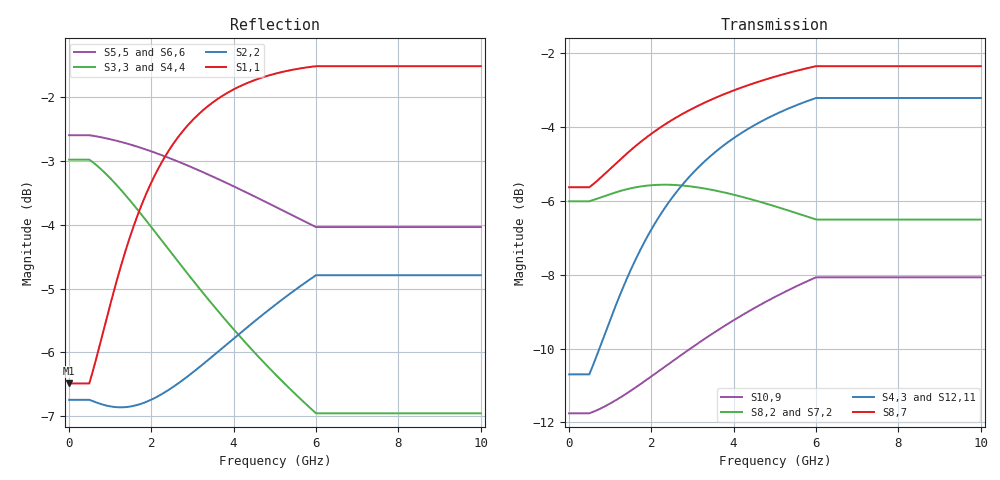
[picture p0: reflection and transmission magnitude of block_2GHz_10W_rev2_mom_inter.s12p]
! Created Wed May 20 10:39:07 2015
# ghz S ma R 50
! 12 Port Network Data from SP1.SP block
! freq  magS1_1  angS1_1  magS1_2  angS1_2  magS1_3  angS1_3  magS1_4  angS1_4
!  magS1_5  angS1_5  magS1_6  angS1_6  magS1_7  angS1_7  magS1_8  angS1_8
!  magS1_9  angS1_9  magS1_10  angS1_10  magS1_11  angS1_11  magS1_12  angS1_12
!  magS2_1  angS2_1  magS2_2  angS2_2  magS2_3  angS2_3  magS2_4  angS2_4
!  magS2_5  angS2_5  magS2_6  angS2_6  magS2_7  angS2_7  magS2_8  angS2_8
!  magS2_9  angS2_9  magS2_10  angS2_10  magS2_11  angS2_11  magS2_12  angS2_12
!  magS3_1  angS3_1  magS3_2  angS3_2  magS3_3  angS3_3  magS3_4  angS3_4
!  magS3_5  angS3_5  magS3_6  angS3_6  magS3_7  angS3_7  magS3_8  angS3_8
!  magS3_9  angS3_9  magS3_10  angS3_10  magS3_11  angS3_11  magS3_12  angS3_12
!  magS4_1  angS4_1  magS4_2  angS4_2  magS4_3  angS4_3  magS4_4  angS4_4
!  magS4_5  angS4_5  magS4_6  angS4_6  magS4_7  angS4_7  magS4_8  angS4_8
!  magS4_9  angS4_9  magS4_10  angS4_10  magS4_11  angS4_11  magS4_12  angS4_12
!  magS5_1  angS5_1  magS5_2  angS5_2  magS5_3  angS5_3  magS5_4  angS5_4
!  magS5_5  angS5_5  magS5_6  angS5_6  magS5_7  angS5_7  magS5_8  angS5_8
!  magS5_9  angS5_9  magS5_10  angS5_10  magS5_11  angS5_11  magS5_12  angS5_12
!  magS6_1  angS6_1  magS6_2  angS6_2  magS6_3  angS6_3  magS6_4  angS6_4
!  magS6_5  angS6_5  magS6_6  angS6_6  magS6_7  angS6_7  magS6_8  angS6_8
!  magS6_9  angS6_9  magS6_10  angS6_10  magS6_11  angS6_11  magS6_12  angS6_12
!  magS7_1  angS7_1  magS7_2  angS7_2  magS7_3  angS7_3  magS7_4  angS7_4
!  magS7_5  angS7_5  magS7_6  angS7_6  magS7_7  angS7_7  magS7_8  angS7_8
!  magS7_9  angS7_9  magS7_10  angS7_10  magS7_11  angS7_11  magS7_12  angS7_12
!  magS8_1  angS8_1  magS8_2  angS8_2  magS8_3  angS8_3  magS8_4  angS8_4
!  magS8_5  angS8_5  magS8_6  angS8_6  magS8_7  angS8_7  magS8_8  angS8_8
!  magS8_9  angS8_9  magS8_10  angS8_10  magS8_11  angS8_11  magS8_12  angS8_12
!  magS9_1  angS9_1  magS9_2  angS9_2  magS9_3  angS9_3  magS9_4  angS9_4
!  magS9_5  angS9_5  magS9_6  angS9_6  magS9_7  angS9_7  magS9_8  angS9_8
!  magS9_9  angS9_9  magS9_10  angS9_10  magS9_11  angS9_11  magS9_12  angS9_12
!  magS10_1  angS10_1  magS10_2  angS10_2  magS10_3  angS10_3  magS10_4  angS10_4
!  magS10_5  angS10_5  magS10_6  angS10_6  magS10_7  angS10_7  magS10_8  angS10_8
!  magS10_9  angS10_9  magS10_10  angS10_10  magS10_11  angS10_11  magS10_12  angS10_12
!  magS11_1  angS11_1  magS11_2  angS11_2  magS11_3  angS11_3  magS11_4  angS11_4
!  magS11_5  angS11_5  magS11_6  angS11_6  magS11_7  angS11_7  magS11_8  angS11_8
!  magS11_9  angS11_9  magS11_10  angS11_10  magS11_11  angS11_11  magS11_12  angS11_12
!  magS12_1  angS12_1  magS12_2  angS12_2  magS12_3  angS12_3  magS12_4  angS12_4
!  magS12_5  angS12_5  magS12_6  angS12_6  magS12_7  angS12_7  magS12_8  angS12_8
!  magS12_9  angS12_9  magS12_10  angS12_10  magS12_11  angS12_11  magS12_12  angS12_12
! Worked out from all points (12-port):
!   1000 points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, 10 MHz to 10 GHz, reference 50 ohm
!   strongest paths, dB at 10 MHz, 2.51 GHz, 5.01 GHz, 7.51 GHz, 10 GHz:
!     S8,7: -5.6, -3.8, -2.6, -2.3, -2.3
!     S4,3: -10.7, -5.9, -3.7, -3.2, -3.2
!     S12,11: -10.7, -5.9, -3.7, -3.2, -3.2
!     S8,2: -6.0, -5.6, -6.1, -6.5, -6.5
!     S7,2: -6.0, -5.6, -6.2, -6.5, -6.5
!     S10,9: -11.8, -10.4, -8.6, -8.1, -8.1
!   lowest |S11| = -6.5 dB at 10 MHz (marker M1), VSWR 2.80, Z = 20.4 + j17.5 ohm
!   |S11| at or under -10 dB: nowhere
